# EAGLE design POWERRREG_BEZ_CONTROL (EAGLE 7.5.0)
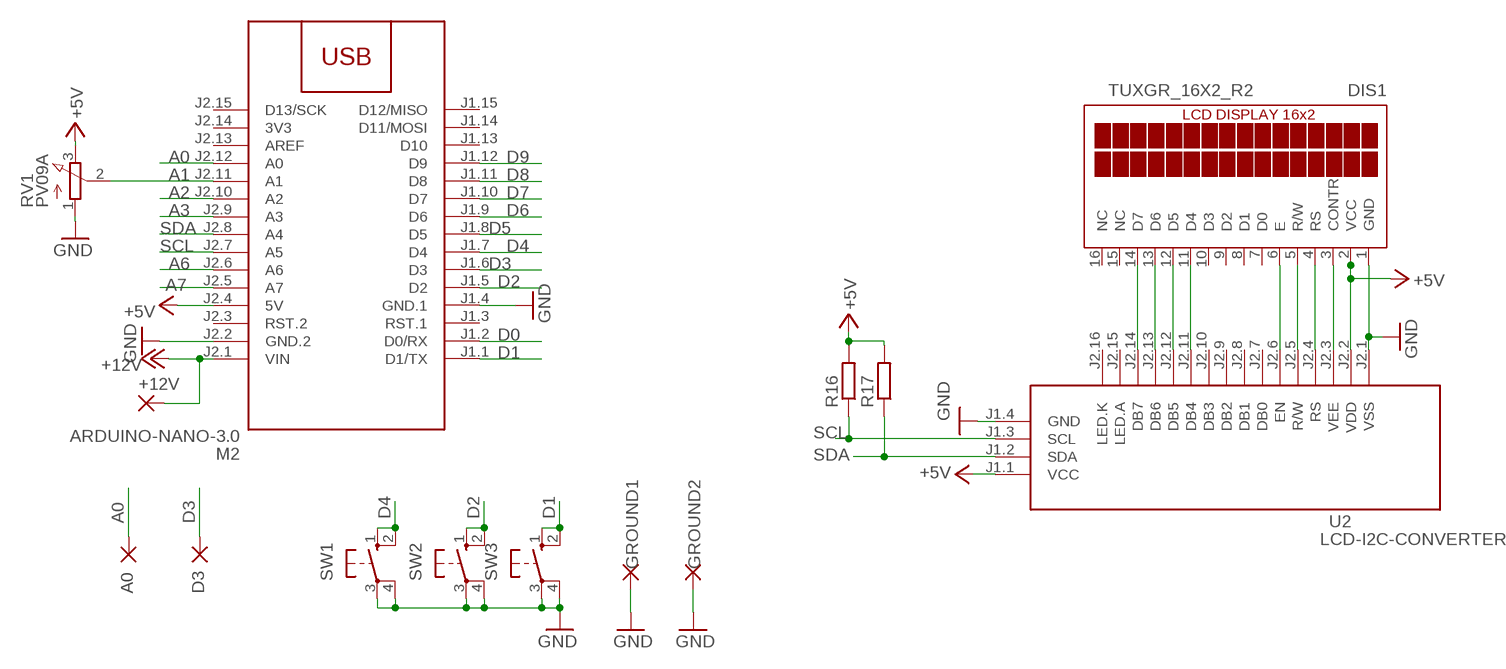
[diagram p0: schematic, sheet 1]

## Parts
+12V  2,54/0,8  [2,54/0,8]
A0  2,54/0,8  [2,54/0,8]
D3  2,54/0,8  [2,54/0,8]
DIS1  TUXGR_16X2_R2  [TUXGR_16X2_R2]
GROUND1  2,54/0,8  [2,54/0,8]
GROUND2  2,54/0,8  [2,54/0,8]
M2  ARDUINO-NANO-3.0  [ARDUINO-NANO-3.0]
R16  R-EU_R1206  [R1206]
R17  R-EU_R1206  [R1206]
RV1  PV09A  [PTV09]
SW1  40-XX  [B3F-40XX]
SW2  40-XX  [B3F-40XX]
SW3  40-XX  [B3F-40XX]
U2  LCD-I2C-CONVERTER  [LCD-I2C-CONVERTER]

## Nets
+5V: DIS1.2(VCC) M2.J2.4(5V) R16.2 R17.2 RV1.3(E) U2.J1.1(VCC) U2.J2.2(VDD)
+12V: +12V.1(P) M2.J2.1(VIN)
A0: A0.1(P) M2.J2.12(A0)
A1: M2.J2.11(A1) RV1.2(S)
A2: M2.J2.10(A2)
A3: M2.J2.9(A3)
A6: M2.J2.6(A6)
A7: M2.J2.5(A7)
D0: M2.J1.2(D0/RX)
D1: M2.J1.1(D1/TX) SW3.1(S) SW3.2(S1)
D2: M2.J1.5(D2) SW2.1(S) SW2.2(S1)
D3: D3.1(P) M2.J1.6(D3)
D4: M2.J1.7(D4) SW1.1(S) SW1.2(S1)
D5: M2.J1.8(D5)
D6: M2.J1.9(D6)
D7: M2.J1.10(D7)
D8: M2.J1.11(D8)
D9: M2.J1.12(D9)
GND: DIS1.1(GND) GROUND1.1(P) GROUND2.1(P) M2.J1.4(GND.1) M2.J2.2(GND.2) RV1.1(A) SW1.3(P) SW1.4(P1) SW2.3(P) SW2.4(P1) SW3.3(P) SW3.4(P1) U2.J1.4(GND) U2.J2.1(VSS)
N$1: DIS1.14(D7) U2.J2.14(DB7)
N$2: DIS1.13(D6) U2.J2.13(DB6)
N$3: DIS1.12(D5) U2.J2.12(DB5)
N$4: DIS1.11(D4) U2.J2.11(DB4)
N$5: DIS1.6(E) U2.J2.6(EN)
N$6: DIS1.5(R/W) U2.J2.5(R/W)
N$7: DIS1.4(RS) U2.J2.4(RS)
N$10: DIS1.3(CONTR) U2.J2.3(VEE)
SCL: M2.J2.7(A5) R16.1 U2.J1.3(SCL)
SDA: M2.J2.8(A4) R17.1 U2.J1.2(SDA)
Unconnected: DIS1.7(D0) DIS1.8(D1) DIS1.9(D2) DIS1.10(D3) DIS1.15(NC) DIS1.16(NC) M2.J1.3(RST.1) M2.J1.13(D10) M2.J1.14(D11/MOSI) M2.J1.15(D12/MISO) M2.J2.3(RST.2) M2.J2.13(AREF) M2.J2.15(D13/SCK) U2.J2.7(DB0) U2.J2.8(DB1) U2.J2.9(DB2) U2.J2.10(DB3) U2.J2.15(LED.A) U2.J2.16(LED.K)

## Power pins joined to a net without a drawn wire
3V3: M2.J2.14(3V3)

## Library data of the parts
+12V A0 D3 GROUND1 GROUND2 = wirepad:2,54/0,8: THROUGH-HOLE PAD
DIS1 = display-lcd:TUXGR_16X2_R2: Tuxgraphics LCD display 16x2 characters reflective, without background light Source: tuxgr_12x2_r2.pdf; OC_FARNELL: unknown; OC_NEWARK: unknown
M2 = diy-modules:ARDUINO-NANO-3.0: Arduino Nano 3.0 and compatible devices More details available here: https://www.arduino.cc/en/Main/ArduinoBoardNano Click here to find device on ebay.com
R16 R17 = rcl:R-EU_: RESISTOR, European symbol
RV1 = pot:PV09A
SW1-SW3 = switch-omron:40-XX: OMRON SWITCH; MF: OMRON COMPONENTS USA; MPN: B3F-4000; OC_FARNELL: 176434; OC_NEWARK: 36K3105
U2 = diy-modules:LCD-I2C-CONVERTER: I2C Bus to 4-Bit Parallel LCD Interface with LED backlight driver

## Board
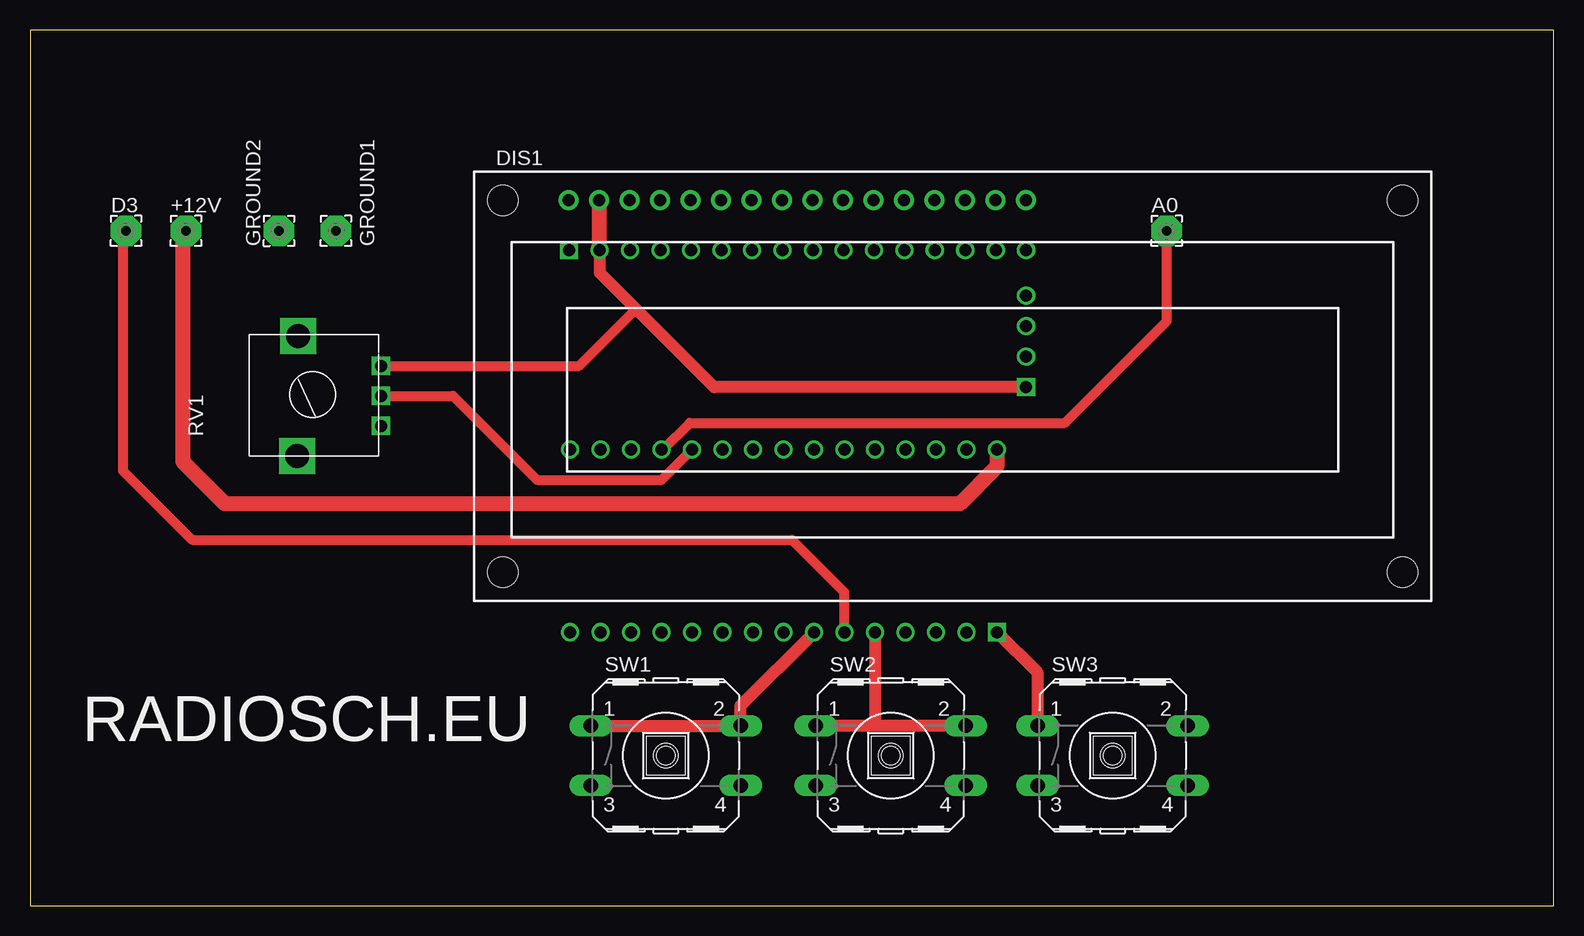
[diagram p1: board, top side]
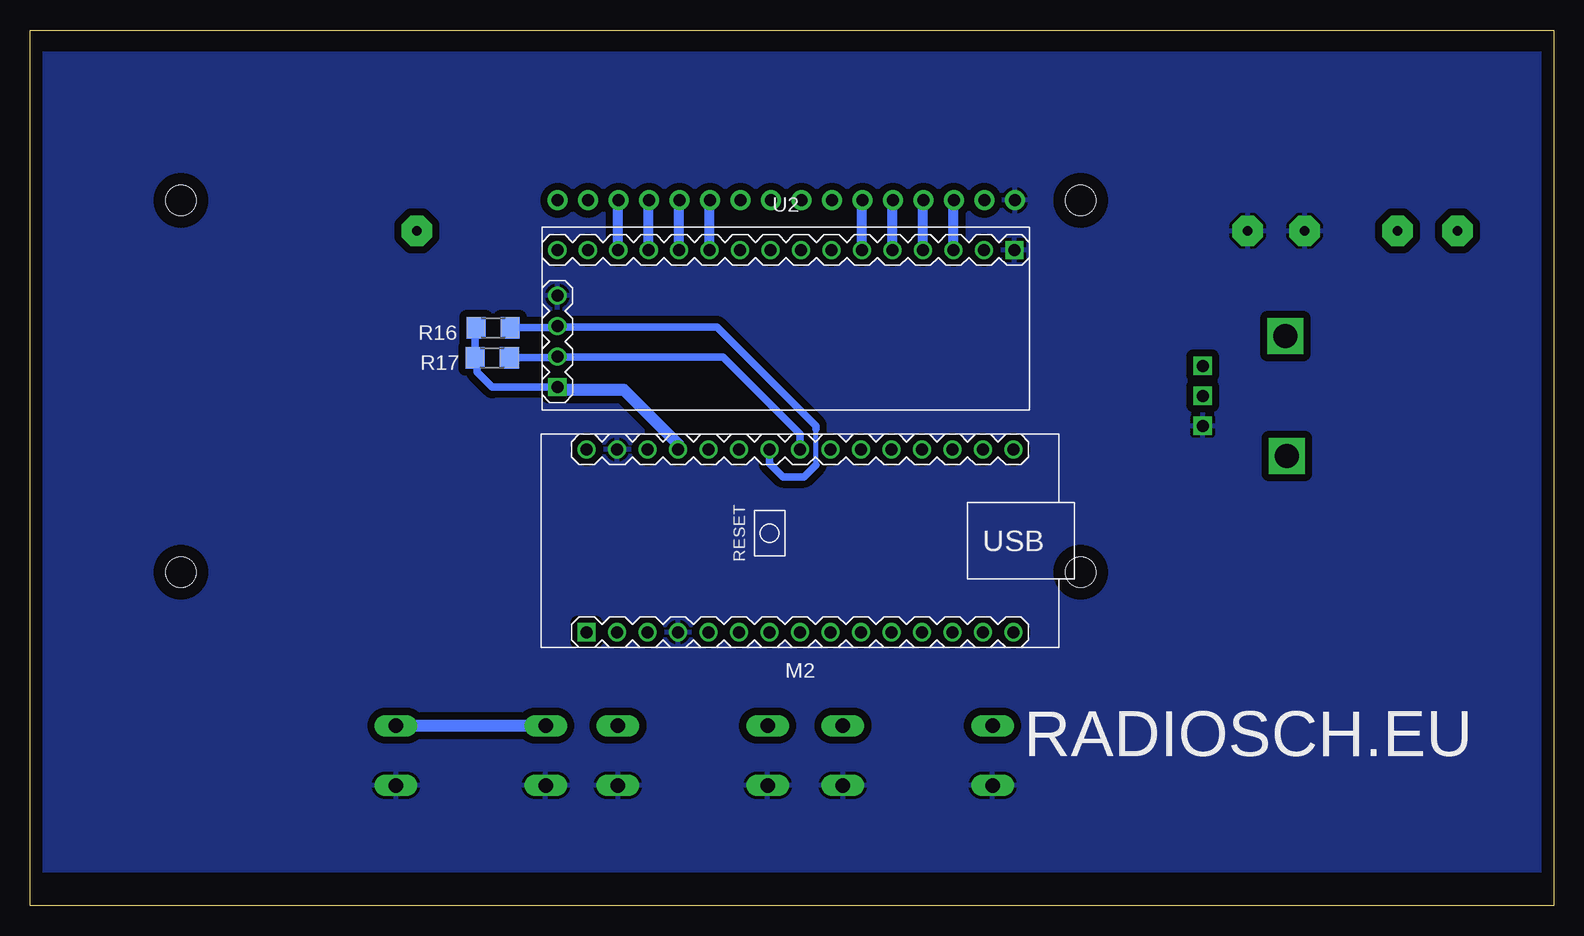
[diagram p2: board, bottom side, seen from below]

Size 127 x 73 mm. Coordinates in mm from the lower left corner, seen from the top.
Outline: 0,0 127,0 127,73 0,73 0,0
Copper layers (1*16): Top 0.035mm / dielectric 1.5mm / Bottom 0.035mm
Design rules "default": minimum track width 10mil, minimum drill 24mil, track to track 8mil, track to pad 8mil, pad to pad 8mil, via to via 8mil, smd to smd 8mil, copper to edge 40mil, drill to drill 8mil, minimum pad ring 10mil, minimum via ring 8mil, stop-mask expansion 4mil, vias tented up to drill 0mil, thermal gap 10mil

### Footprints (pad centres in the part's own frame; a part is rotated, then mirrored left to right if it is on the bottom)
2,54/0,8 = drill 0.813 pad 2.54 octagon: 1 0,0
TUXGR_16X2_R2 = drill 1 pad 1.676: 1 -32,15.5; 2 -29.46,15.5; 3 -26.92,15.5; 4 -24.38,15.5; 5 -21.84,15.5; 6 -19.3,15.5; 7 -16.76,15.5; 8 -14.22,15.5; 9 -11.68,15.5; 10 -9.14,15.5; 11 -6.6,15.5; 12 -4.06,15.5; 13 -1.52,15.5; 14 1.02,15.5; 15 3.56,15.5; 16 6.1,15.5 | hole 2.5: -37.5,-15.5; 37.5,-15.5; -37.5,15.5; 37.5,15.5
ARDUINO-NANO-3.0 = drill 1 square: J1.1 17.78,7.62 | drill 1: J1.2 15.24,7.62; J1.3 12.7,7.62; J1.4 10.16,7.62; J1.5 7.62,7.62; J1.6 5.08,7.62; J1.7 2.54,7.62; J1.8 0,7.62; J1.9 -2.54,7.62; J1.10 -5.08,7.62; J1.11 -7.62,7.62; J1.12 -10.16,7.62; J1.13 -12.7,7.62; J1.14 -15.24,7.62; J1.15 -17.78,7.62; J2.1 17.78,-7.62; J2.2 15.24,-7.62; J2.3 12.7,-7.62; J2.4 10.16,-7.62; J2.5 7.62,-7.62; J2.6 5.08,-7.62; J2.7 2.54,-7.62; J2.8 0,-7.62; J2.9 -2.54,-7.62; J2.10 -5.08,-7.62; J2.11 -7.62,-7.62; J2.12 -10.16,-7.62; J2.13 -12.7,-7.62; J2.14 -15.24,-7.62; J2.15 -17.78,-7.62
R1206 = smd 1.6 x 1.803: 1 -1.422,0; 2 1.422,0
PTV09 = drill 1 square: 1 -2.5,0; 2 0,0; 3 2.5,0 | drill 2 square: P$4 -5,7; P$5 5,6.9
B3F-40XX = drill 1.194 long: 1 -6.248,2.489; 2 6.248,2.489; 3 -6.248,-2.489; 4 6.248,-2.489
LCD-I2C-CONVERTER = drill 1 square: J1.1 -19.05,-5.08; J2.1 19.05,6.35 | drill 1: J1.2 -19.05,-2.54; J1.3 -19.05,0; J1.4 -19.05,2.54; J2.2 16.51,6.35; J2.3 13.97,6.35; J2.4 11.43,6.35; J2.5 8.89,6.35; J2.6 6.35,6.35; J2.7 3.81,6.35; J2.8 1.27,6.35; J2.9 -1.27,6.35; J2.10 -3.81,6.35; J2.11 -6.35,6.35; J2.12 -8.89,6.35; J2.13 -11.43,6.35; J2.14 -13.97,6.35; J2.15 -16.51,6.35; J2.16 -19.05,6.35

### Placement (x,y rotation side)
+12V  13,56.25 0 top
A0  94.75,56.25 0 top
D3  8,56.25 0 top
DIS1  76.91,43.3 0 top
GROUND1  25.5,56.25 0 top
GROUND2  20.75,56.25 90 top
M2  62.81,30.41 180 bottom
R16  88.39,48.18 180 bottom
R17  88.47,45.68 180 bottom
RV1  29.25,42.5 90 top
SW1  53,12.5 0 top
SW2  71.75,12.5 0 top
SW3  90.25,12.5 0 top
U2  63.99,48.3 0 bottom

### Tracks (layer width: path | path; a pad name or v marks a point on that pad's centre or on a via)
+5V
  Top 0.813: RV1.3 45.75,45 50.5,49.75
  Top 1.016: U2.J1.1 57.03,43.22 50.5,49.75 47.5,52.75 47.5,54.63 U2.J2.2
  Top 1.27: U2.J2.2 47.48,58.77 DIS1.2
  Bottom 0.61: U2.J1.1 88.47,43.22 89.75,44.5 89.75,45.54 R17.2 89.89,48.1 R16.2
  Bottom 1.016: M2.J2.4 72.97,38.47 77.5,43 82.82,43 U2.J1.1
+12V
  Top 1.27: M2.J2.1 80.59,36.59 77.5,33.5 16.25,33.5 12.75,37 12.75,56 +12V.1
A0
  Top 0.813: M2.J2.12 52.78,38.03 55,40.25 86.25,40.25 94.75,48.75 A0.1
A1
  Top 0.813: RV1.2 35.25,42.5 42.25,35.5 52.66,35.5 M2.J2.11
D1
  Top 1.016: SW3.1 84,19.38 M2.J1.1
  Bottom 1.016: SW3.1 SW3.2
D2
  Top 1.016: SW2.2 70.75,14.99 | 70.75,14.99 SW2.1 | M2.J1.5 70.43,15.31 70.75,14.99
D3
  Top 0.813: M2.J1.6 67.89,26.11 63.5,30.5 13.5,30.5 7.75,36.25 7.75,56 D3.1
D4
  Top 1.016: M2.J1.7 59.25,16.69 SW1.2 SW1.1
GND
  pour Bottom (isolate 0.61): 1,71 126,71 126,3 1,3
N$1
  Bottom 0.813: U2.J2.14 77.96,58.77 DIS1.14
N$2
  Bottom 0.813: U2.J2.13 75.42,58.77 DIS1.13
N$3
  Bottom 0.813: U2.J2.12 72.88,58.77 DIS1.12
N$4
  Bottom 0.813: U2.J2.11 70.34,58.77 DIS1.11
N$5
  Bottom 0.813: U2.J2.6 57.64,58.77 DIS1.6
N$6
  Bottom 0.813: U2.J2.5 55.1,58.77 DIS1.5
N$7
  Bottom 0.813: U2.J2.4 52.56,58.77 DIS1.4
N$10
  Bottom 0.813: U2.J2.3 50.02,58.77 DIS1.3
SCL
  Bottom 0.406: 61.5,36.75 61.5,39.75
  Bottom 0.61: M2.J2.7 65.35,36.85 64.25,35.75 62.5,35.75 61.5,36.75 | 61.5,39.75 61.5,40 69.75,48.25 82.99,48.25 U2.J1.3 83.16,48.18 R16.1
SDA
  Bottom 0.61: M2.J2.8 62.81,39.31 69.25,45.75 U2.J1.2 83.12,45.68 R17.1

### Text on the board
tPlace: RADIOSCH.EU
bPlace: RADIOSCH.EU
